(* Logix 5000 AddOnInstructionDefinition export AMCI_3601_AOP_Registration_CCW; software revision 20.03 *)

ADD_ON_INSTRUCTION AMCI_3601_AOP_Registration_CCW   (* revision 0.0, vendor AMCI, ExecuteEnableInFalse *)
// Revision note:
// 3/2020: Version 0 is the initial release
VAR_INPUT
   Axis_Status_Bits : INT; {required}
   _0_normal_1_S_Curve_Acceleration : BOOL;
   _0_Triangular_1_Trapezoidal_S_Curve : BOOL;
   Target_Position : DINT; {required}
   Programmed_Speed : DINT; {required}
   Acceleration : INT; {required}
   Deceleration : INT; {required}
END_VAR
VAR_OUTPUT
   EN : BOOL; {access Read Only, visible}
   Registration_Move_CCW_Occurring : BOOL; {access Read Only, visible}
   ER : BOOL; {access Read Only, visible}
END_VAR
VAR_IN_OUT
   AMCI_3601_output_data : AM:1769_3601:O:0; {required}
END_VAR
VAR
   Upper_Result_X_1000 : DINT;
   command_data_block : INT[10];
        [0]   // Command Bits MSW
        [1]   // Command Bits LSW
        [2]   // Upper Target Position
        [3]   // Lower Target Position
        [4]   // Upper Programmed Speed
        [5]   // Lower Programmed Speed
END_VAR

ROUTINE EnableInFalse   (* ladder *)
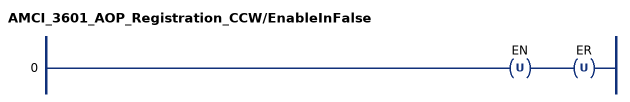
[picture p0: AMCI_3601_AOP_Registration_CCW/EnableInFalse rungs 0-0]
   0: OTU(EN)OTU(ER);
END_ROUTINE

ROUTINE Logic   (* ladder *)
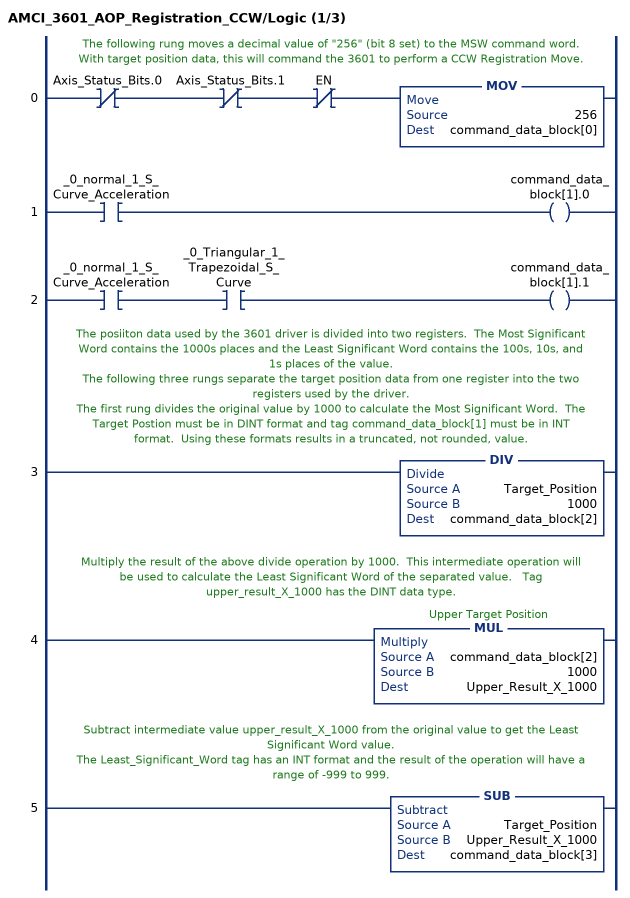
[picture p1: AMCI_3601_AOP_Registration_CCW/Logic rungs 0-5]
   // The following rung moves a decimal value of "256" (bit 8 set) to the MSW command word.  With target position data, this will command the 3601 to perform a CCW Registration Move.
   0: XIO(Axis_Status_Bits.0)XIO(Axis_Status_Bits.1)XIO(EN)MOV(256,command_data_block[0]);
   1: XIC(_0_normal_1_S_Curve_Acceleration)OTE(command_data_block[1].0);
   2: XIC(_0_normal_1_S_Curve_Acceleration)XIC(_0_Triangular_1_Trapezoidal_S_Curve)OTE(command_data_block[1].1);
   // The posiiton data used by the 3601 driver is divided into two registers.  The Most Significant Word contains the 1000s places and the Least Significant Word contains the 100s, 10s, and 1s places of the value.
   // The following three rungs separate the target position data from one register into the two registers used by the driver.
   // The first rung divides the original value by 1000 to calculate the Most Significant Word.  The Target Postion must be in DINT format and tag command_data_block[1] must be in INT format.  Using these formats results in a truncated, not rounded, value.
   3: DIV(Target_Position,1000,command_data_block[2]);
   // Multiply the result of the above divide operation by 1000.  This intermediate operation will be used to calculate the Least Significant Word of the separated value.   Tag upper_result_X_1000 has the DINT data type.
   4: MUL(command_data_block[2],1000,Upper_Result_X_1000);
   // Subtract intermediate value upper_result_X_1000 from the original value to get the Least Significant Word value.
   // The Least_Significant_Word tag has an INT format and the result of the operation will have a range of -999 to 999.
   5: SUB(Target_Position,Upper_Result_X_1000,command_data_block[3]);
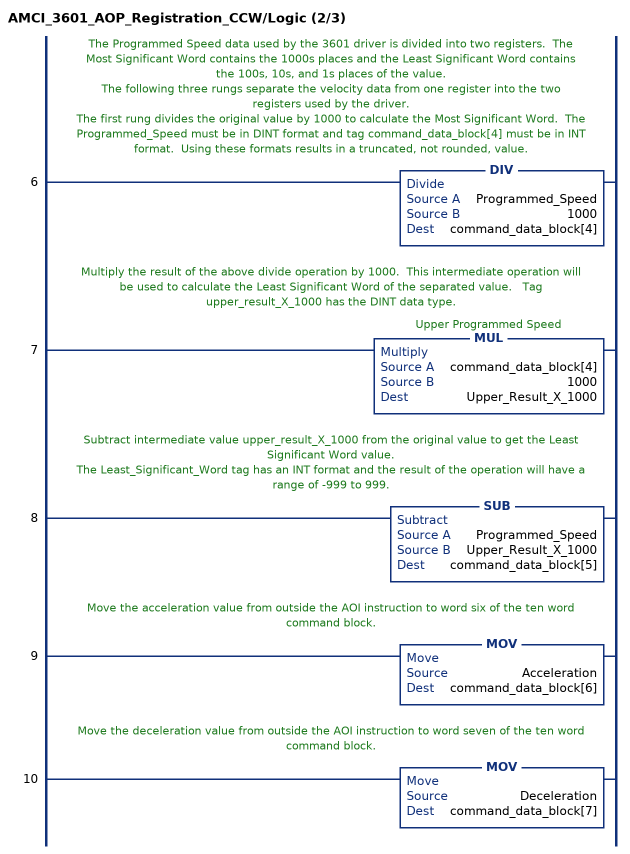
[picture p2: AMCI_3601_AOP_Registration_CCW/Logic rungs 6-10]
   // The Programmed Speed data used by the 3601 driver is divided into two registers.  The Most Significant Word contains the 1000s places and the Least Significant Word contains the 100s, 10s, and 1s places of the value.
   // The following three rungs separate the velocity data from one register into the two registers used by the driver.
   // The first rung divides the original value by 1000 to calculate the Most Significant Word.  The Programmed_Speed must be in DINT format and tag command_data_block[4] must be in INT format.  Using these formats results in a truncated, not rounded, value.
   6: DIV(Programmed_Speed,1000,command_data_block[4]);
   // Multiply the result of the above divide operation by 1000.  This intermediate operation will be used to calculate the Least Significant Word of the separated value.   Tag upper_result_X_1000 has the DINT data type.
   7: MUL(command_data_block[4],1000,Upper_Result_X_1000);
   // Subtract intermediate value upper_result_X_1000 from the original value to get the Least Significant Word value.
   // The Least_Significant_Word tag has an INT format and the result of the operation will have a range of -999 to 999.
   8: SUB(Programmed_Speed,Upper_Result_X_1000,command_data_block[5]);
   // Move the acceleration value from outside the AOI instruction to word six of the ten word command block.
   9: MOV(Acceleration,command_data_block[6]);
   // Move the deceleration value from outside the AOI instruction to word seven of the ten word command block.
   10: MOV(Deceleration,command_data_block[7]);
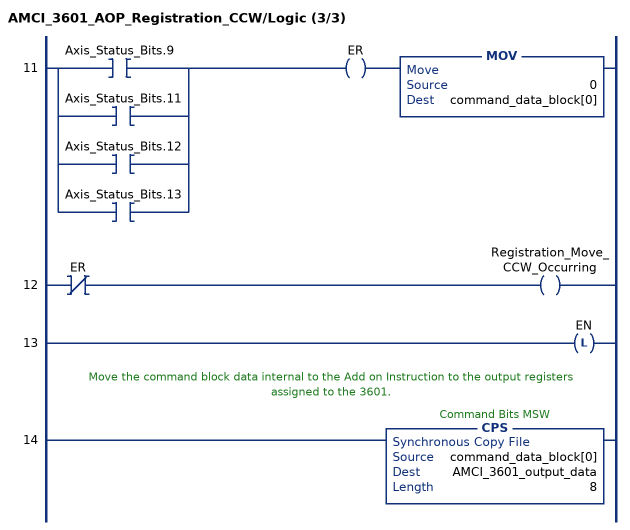
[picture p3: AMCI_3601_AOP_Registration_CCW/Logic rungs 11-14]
   11: [XIC(Axis_Status_Bits.9) ,XIC(Axis_Status_Bits.11) ,XIC(Axis_Status_Bits.12) ,XIC(Axis_Status_Bits.13) ]OTE(ER)MOV(0,command_data_block[0]);
   12: XIO(ER)OTE(Registration_Move_CCW_Occurring);
   13: OTL(EN);
   // Move the command block data internal to the Add on Instruction to the output registers assigned to the 3601.
   14: CPS(command_data_block[0],AMCI_3601_output_data,8);
END_ROUTINE
END_ADD_ON_INSTRUCTION
